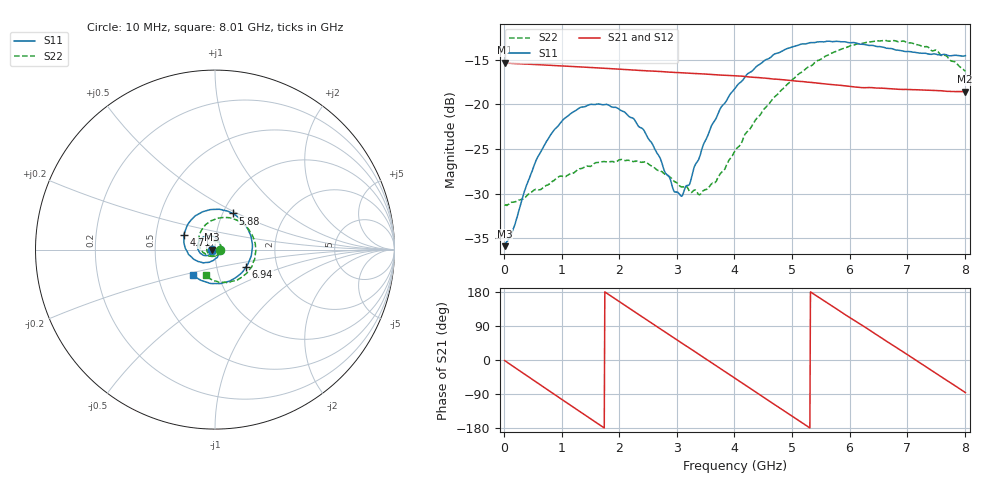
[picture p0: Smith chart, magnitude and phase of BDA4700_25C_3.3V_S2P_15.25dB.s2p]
!Agilent Technologies,E5071B,MY42404982,A.09.10
!Date: Mon Oct 20 18:09:26 2025
!Data & Calibration Information:
!Freq	S11:SOLT2(ON)	S21:SOLT2(ON)	S12:SOLT2(ON)	S22:SOLT2(ON)
# Hz S RI R 50
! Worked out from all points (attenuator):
!   801 points, 10 MHz to 8.01 GHz, reference 50 ohm
!   highest |S21| = -15.34 dB at 10 MHz (marker M1); lowest = -18.6 dB at 8 GHz (marker M2)
!   lowest |S11| = -35.9 dB at 10 MHz (marker M3), VSWR 1.03, Z = 48.4 - j0.111 ohm
!   |S11| at or under -10 dB: start of sweep to end of sweep
!   |S22| runs from -31.3 to -12.8 dB; largest |S21 - S12| = 0.002
!   S11 on the Smith chart (normalised r, x): 10 MHz: 0.97, -0.00; 4.71 GHz: 0.70, +0.12; 5.88 GHz: 1.11, +0.47; 6.94 GHz: 1.39, -0.27; 8.01 GHz: 0.75, -0.22
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1e7  -0.016 -0.00114  0.1709 -0.0037  0.1708 -0.0039  0.0274 -0.000994
1.5e8  -0.0172 -0.00959  0.1628 -0.0466  0.1629 -0.0466  0.0272 -0.00766
7e8  -0.0485 -0.0336  0.0488 -0.1588  0.049 -0.1587  0.00429 -0.0344
1.03e9  -0.0789 -0.023  -0.0474 -0.157  -0.0473 -0.157  -0.0204 -0.0337
1.35e9  -0.0964 0.00662  -0.1232 -0.1051  -0.1232 -0.1052  -0.0412 -0.0147
2.08e9  -0.0497 0.0763  -0.1302 0.0874  -0.1303 0.0875  -0.0243 0.042
2.42e9  -0.00487 0.0721  -0.0573 0.1435  -0.0572 0.1435  0.00609 0.047
2.68e9  0.0219 0.0472  0.0118 0.1525  0.0116 0.1524  0.0249 0.0346
2.95e9  0.0313 0.00934  0.0792 0.1287  0.0789 0.1284  0.0343 0.0141
3.09e9  0.0285 -0.0114  0.1078 0.1047  0.1068 0.1053  0.0344 0.000794
3.41e9  -0.000434 -0.0524  0.1449 0.0315  0.1451 0.0315  0.0193 -0.0248
3.75e9  -0.0585 -0.0733  0.1355 -0.0544  0.1356 -0.0544  -0.0139 -0.0383
4.01e9  -0.1075 -0.0595  0.0964 -0.1078  0.0966 -0.1075  -0.045 -0.0313
4.71e9  -0.1738 0.0821  -0.067 -0.1212  -0.0665 -0.1216  -0.0907 0.0639
5.35e9  -0.0609 0.2132  -0.1323 0.00745  -0.1323 0.00672  -0.0076 0.1654
5.88e9  0.0986 0.2013  -0.0715 0.1055  -0.0715 0.1052  0.1251 0.1625
6.27e9  0.1836 0.1139  0.00757 0.1238  0.00924 0.1233  0.2034 0.0872
6.68e9  0.205 -0.0173  0.0854 0.0876  0.0857 0.0875  0.2249 -0.0256
6.94e9  0.1744 -0.0946  0.1135 0.0423  0.1138 0.0416  0.2039 -0.097
7.47e9  0.0338 -0.1887  0.1013 -0.0637  0.1012 -0.064  0.0804 -0.1835
8e9  -0.122 -0.1415  0.0101 -0.1173  0.0104 -0.1174  -0.0506 -0.1457
8.01e9  -0.1244 -0.1401  0.00804 -0.1175  0.00851 -0.1176  -0.0526 -0.1437
